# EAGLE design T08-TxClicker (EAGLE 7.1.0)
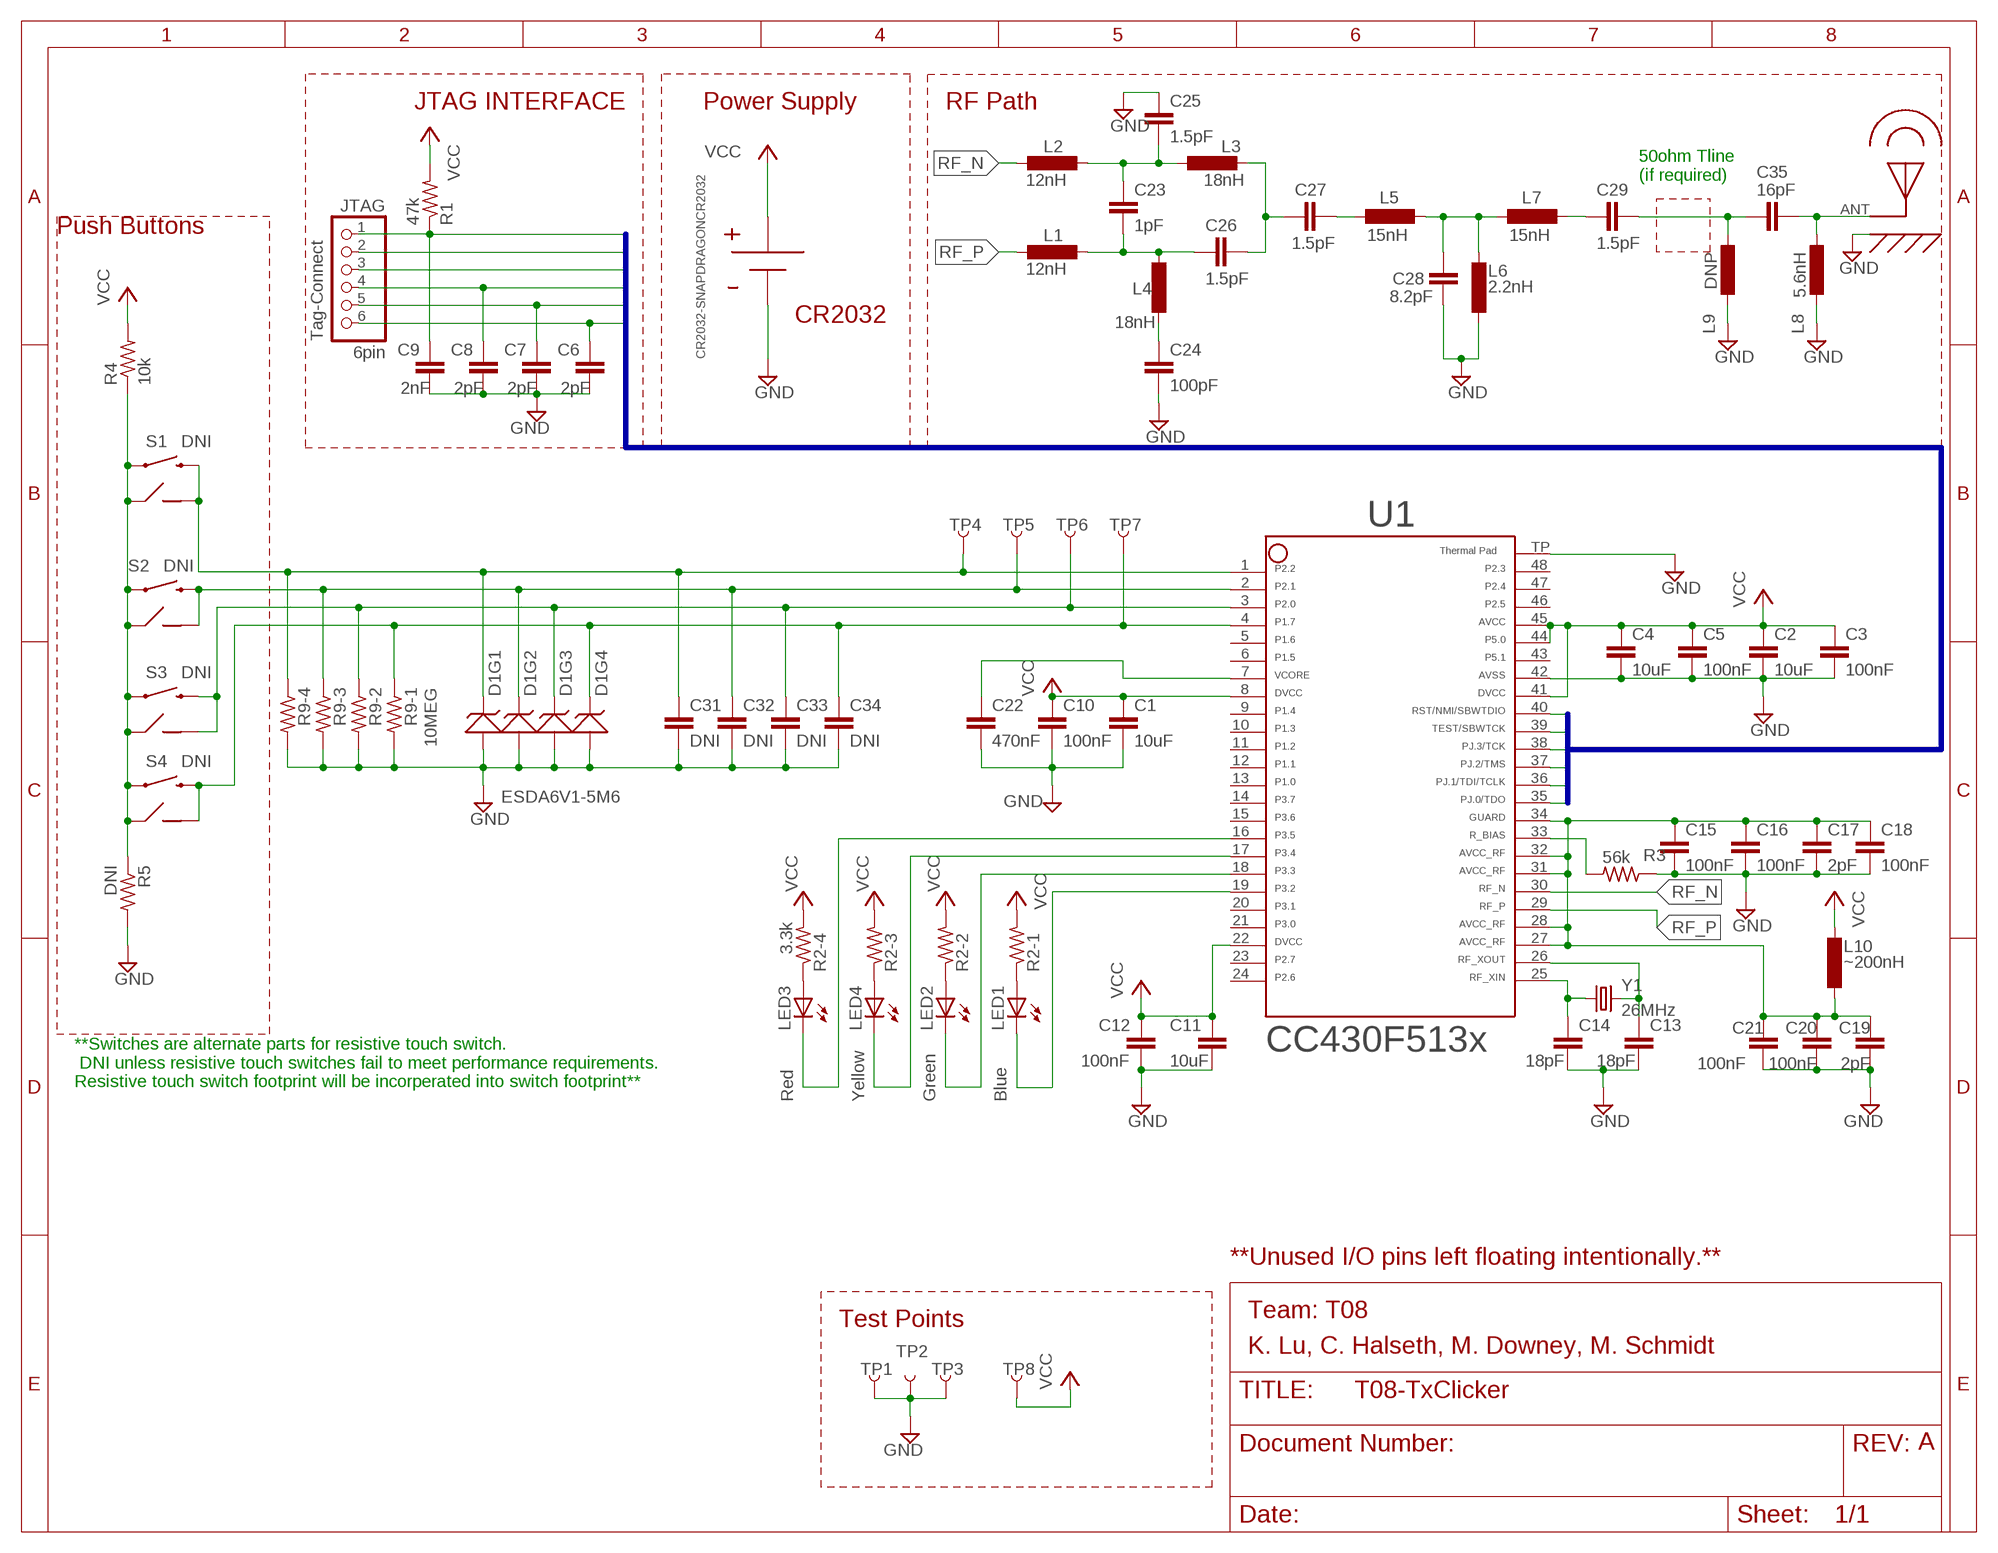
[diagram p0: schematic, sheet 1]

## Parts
C1  10uF  C-EUC0805  [C0805]
C2  10uF  C-EUC0805  [C0805]
C3  100nF  C-EUC0603  [C0603]
C4  10uF  C-EUC0805  [C0805]
C5  100nF  C-EUC0603  [C0603]
C6  2pF  C0603  [C0603]
C7  2pF  C0603  [C0603]
C8  2pF  C0603  [C0603]
C9  2nF  C0603  [C0603]
C10  100nF  C-EUC0603  [C0603]
C11  10uF  C-EUC0805  [C0805]
C12  100nF  C-EUC0603  [C0603]
C13  18pF  C-EUC0402  [C0402]
C14  18pF  C-EUC0402  [C0402]
C15  100nF  C-EUC0603  [C0603]
C16  100nF  C-EUC0603  [C0603]
C17  2pF  C-EUC0603  [C0603]
C18  100nF  C-EUC0603  [C0603]
C19  2pF  C-EUC0603  [C0603]
C20  100nF  C-EUC0603  [C0603]
C21  100nF  C-EUC0603  [C0603]
C22  470nF  C-EUC0603  [C0603]
C23  1pF  C-EUC0402  [C0402]
C24  100pF  C-EUC0402  [C0402]
C25  1.5pF  C-EUC0402  [C0402]
C26  1.5pF  C-EUC0402  [C0402]
C27  1.5pF  C-EUC0402  [C0402]
C28  8.2pF  C-EUC0402  [C0402]
C29  1.5pF  C-EUC0402  [C0402]
C31  DNI  C-EUC0603  [C0603]
C32  DNI  C-EUC0603  [C0603]
C33  DNI  C-EUC0603  [C0603]
C34  DNI  C-EUC0603  [C0603]
C35  16pF  C-EUC0402  [C0402]
D1  ESDA6V1-5M6  [5X-TVS]
JTAG  6pin  PINHD-1X6  [1X06]
L1  12nH  LL0603  [L0603]
L2  12nH  LL0603  [L0603]
L3  18nH  LL0603  [L0603]
L4  18nH  LL0603  [L0603]
L5  15nH  LL0603  [L0603]
L6  2.2nH  LL0603  [L0603]
L7  15nH  LL0603  [L0603]
L8  5.6nH  LL0603  [L0603]
L9  DNP  LL0603  [L0603]
L10  ~200nH  LL0402  [L0402]
LED1  Blue  LEDCHIP-LED0603  [CHIP-LED0603]
LED2  Green  LEDCHIP-LED0603  [CHIP-LED0603]
LED3  Red  LEDCHIP-LED0603  [CHIP-LED0603]
LED4  Yellow  LEDCHIP-LED0603  [CHIP-LED0603]
R1  47k  R-US_R0603  [R0603]
R2  3.3k  R603X42012  [2012(4_RES)]
R3  56k  R-US_R0603  [R0603]
R4  10k  R-US_R0603  [R0603]
R5  DNI  R-US_R0603  [R0603]
R9  10MEG  R603X42012  [2012(4_RES)]
S1  SWITCH-MOMENTARY-212MM  [TACTILE-PTH-12MM]
S2  SWITCH-MOMENTARY-212MM  [TACTILE-PTH-12MM]
S3  SWITCH-MOMENTARY-212MM  [TACTILE-PTH-12MM]
S4  SWITCH-MOMENTARY-212MM  [TACTILE-PTH-12MM]
TP1  TEST-POINT3  [PAD.03X.03]
TP2  TEST-POINT3  [PAD.03X.03]
TP3  TEST-POINT3  [PAD.03X.03]
TP4  TEST-POINT3  [PAD.03X.03]
TP5  TEST-POINT3  [PAD.03X.03]
TP6  TEST-POINT3  [PAD.03X.03]
TP7  TEST-POINT3  [PAD.03X.03]
TP8  TEST-POINT3  [PAD.03X.03]
U1  CC430F513X---RGZ48  [RGZ48]
U$1  TOUCH-PAD  [TOUCH-PAD]
U$2  CR2032-SNAPDRAGONCR2032  [CR2032-SNAPDRAGON]
U$3  TOUCH-PAD  [TOUCH-PAD]
U$4  TOUCH-PAD  [TOUCH-PAD]
U$5  TOUCH-PAD  [TOUCH-PAD]
U$7  PCB_ANTENNA_915MHZOSHP  [PCB_ANTENNA_915MHZ]
Y1  26MHz  CRYSTALTXC-7A  [CRYSTAL-TXC-7A]

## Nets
GND: C1.2 C2.2 C3.2 C4.2 C5.2 C6.2 C7.2 C8.2 C9.2 C10.2 C11.2 C12.2 C13.2 C14.2 C15.2 C16.2 C17.2 C18.2 C19.2 C20.2 C21.2 C22.2 C24.2 C25.1 C28.1 C31.2 C32.2 C33.2 C34.2 D1.2 L6.2 L8.1 L9.1 R3.1 R5.2 R9.2 R9.4 R9.6 R9.8 TP1.P$1 TP2.P$1 TP3.P$1 U1.42 U1.TP U$2.V- U$7.GPLANE
N$1: C23.2 C26.2 L1.1 L4.1
N$2: C23.1 C25.2 L2.1 L3.2
N$3: C26.1 C27.1 L3.1
N$4: C24.1 L4.2
N$5: C27.2 L5.1
N$6: C28.2 L5.2 L6.1 L7.1
N$7: C29.1 C35.2 L9.2
N$8: C29.2 L7.2
N$9: C15.1 C16.1 C17.1 C18.1 C19.1 C20.1 C21.1 L10.P$2 U1.27 U1.28 U1.31 U1.32 U1.34
N$10: C35.1 L8.2 U$7.ANT
N$18: LED1.A R2.1
N$20: R4.1 R5.1 S1.1 S2.1 S3.1 S4.1 U$1.P$1 U$1.P$2 U$1.P$3 U$1.P$4 U$3.P$1 U$3.P$2 U$3.P$3 U$3.P$4 U$4.P$1 U$4.P$2 U$4.P$3 U$4.P$4 U$5.P$1 U$5.P$2 U$5.P$3 U$5.P$4
N$21: LED3.A R2.7
N$23: LED4.A R2.5
N$24: LED2.A R2.3
P1.7: C34.1 D1.5 R9.1 S4.3 TP7.P$1 U1.4 U$1.VCC
P2.0: C33.1 D1.4 R9.3 S3.3 TP6.P$1 U1.3 U$3.VCC
P2.1: C32.1 D1.3 R9.5 S2.3 TP5.P$1 U1.2 U$4.VCC
P2.2: C31.1 D1.1 R9.7 S1.3 TP4.P$1 U1.1 U$5.VCC
P3.2: LED1.C U1.19
P3.3: LED2.C U1.18
P3.4: LED4.C U1.17
P3.5: LED3.C U1.16
PJ.0/TDO: C6.1 JTAG.6 U1.35
PJ.1/TDI/TCLK: C7.1 JTAG.5 U1.36
PJ.2/TMS: C8.1 JTAG.4 U1.37
PJ.3/TCK: JTAG.3 U1.38
R_BIAS: R3.2 U1.33
RF_N: L2.2 U1.30
RF_P: L1.2 U1.29
RF_XIN: C14.1 U1.25 Y1.P$1
RF_XOUT: C13.1 U1.26 Y1.P$2
RST/NMI/SBWTDIO: C9.1 JTAG.1 R1.1 U1.40
TEST/SBWTCK: JTAG.2 U1.39
VCC: C1.1 C2.1 C3.1 C4.1 C5.1 C10.1 C11.1 C12.1 L10.P$1 R1.2 R2.2 R2.4 R2.6 R2.8 R4.2 TP8.P$1 U1.8 U1.22 U1.41 U1.44 U1.45 U$2.V+
VCORE: C22.1 U1.7
Unconnected: D1.6 U1.5 U1.6 U1.9 U1.10 U1.11 U1.12 U1.13 U1.14 U1.15 U1.20 U1.21 U1.23 U1.24 U1.43 U1.46 U1.47 U1.48

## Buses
PJ.0/TDO,PJ.1/TDI/TCLK,PJ.2/TMS,PJ.3/TCK,TEST/SBWTCK,RST/NMI/SBWTDIO

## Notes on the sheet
- JTAG INTERFACE | Power Supply | RF Path
- 50ohm Tline
  (if required)
- Push Buttons
- CR2032
- Tag-Connect
- DNI
- DNI
- DNI
- DNI
- **Switches are alternate parts for resistive touch switch.
   DNI unless resistive touch switches fail to meet performance requirements.
  Resistive touch switch footprint will be incorperated into switch footprint**
- **Unused I/O pins left floating intentionally.**
- Team: T08
- Team: T08 | Team: T08 | Team: T08 | Team: T08
- Test Points
- K. Lu, C. Halseth, M. Downey, M. Schmidt
- A

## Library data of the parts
C1-C5 C10-C29 C31-C35 = rcl:C-EU: CAPACITOR, European symbol
C6-C9 = rcl-amber:C
D1 = TVS:ESDA6V1-5M6
JTAG = adafruit:PINHD-1X6: PIN HEADER
L1-L10 = rcl-amber:L
LED1-LED4 = adafruit:LED: LED
R1 R3-R5 = rcl:R-US_: RESISTOR, American symbol
R2 R9 = QuadResistor:R603X4: Quad resistor package 0603
S1-S4 = SparkFun-Electromechanical:SWITCH-MOMENTARY-2: Various NO switches- pushbuttons, reed, etc; PROD_ID: SWCH-09185
TP1-TP8 = SparkFun-Passives:TEST-POINT: Bare copper test points for troubleshooting or ICT
U1 = TI_MSP430_v16_truncated:CC430F513X---RGZ48: ***CC430F513X***RGZ48 ** ** Rev 1.0 ** 06/2010 * http://focus.ti.com/docs/prod/folders/print/cc430f5137.html
U$1 U$3-U$5 = TouchPad:TOUCH-PAD
U$2 = CR2032-SnapDragon:CR2032-SNAPDRAGON: HOLDER SNAP DRAGON CR2032 SMD
U$7 = PCB_Antenna_915MHz-halseth:PCB_ANTENNA_915MHZ
Y1 = SparkFun-FreqCtrl:CRYSTAL: Various standard crystals. Proven footprints. Spark Fun Electronics SKU : COM-00534

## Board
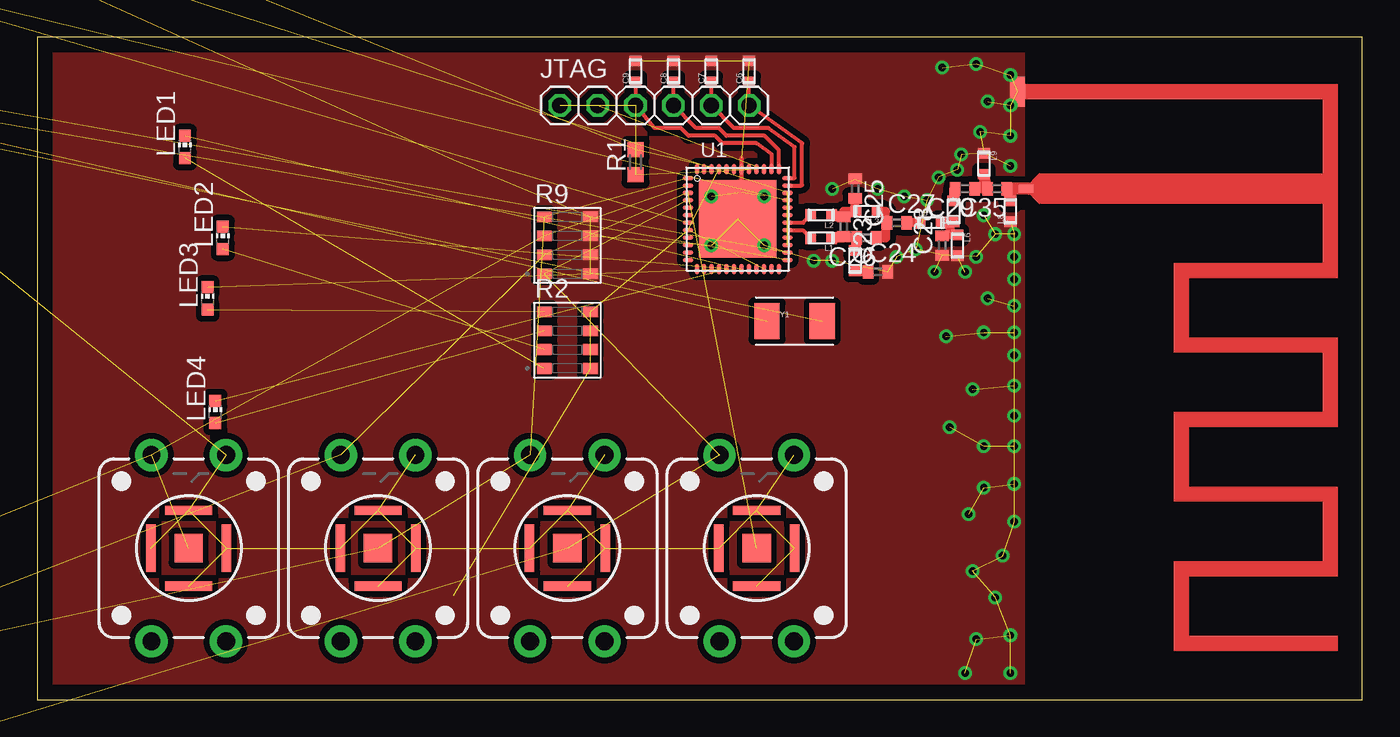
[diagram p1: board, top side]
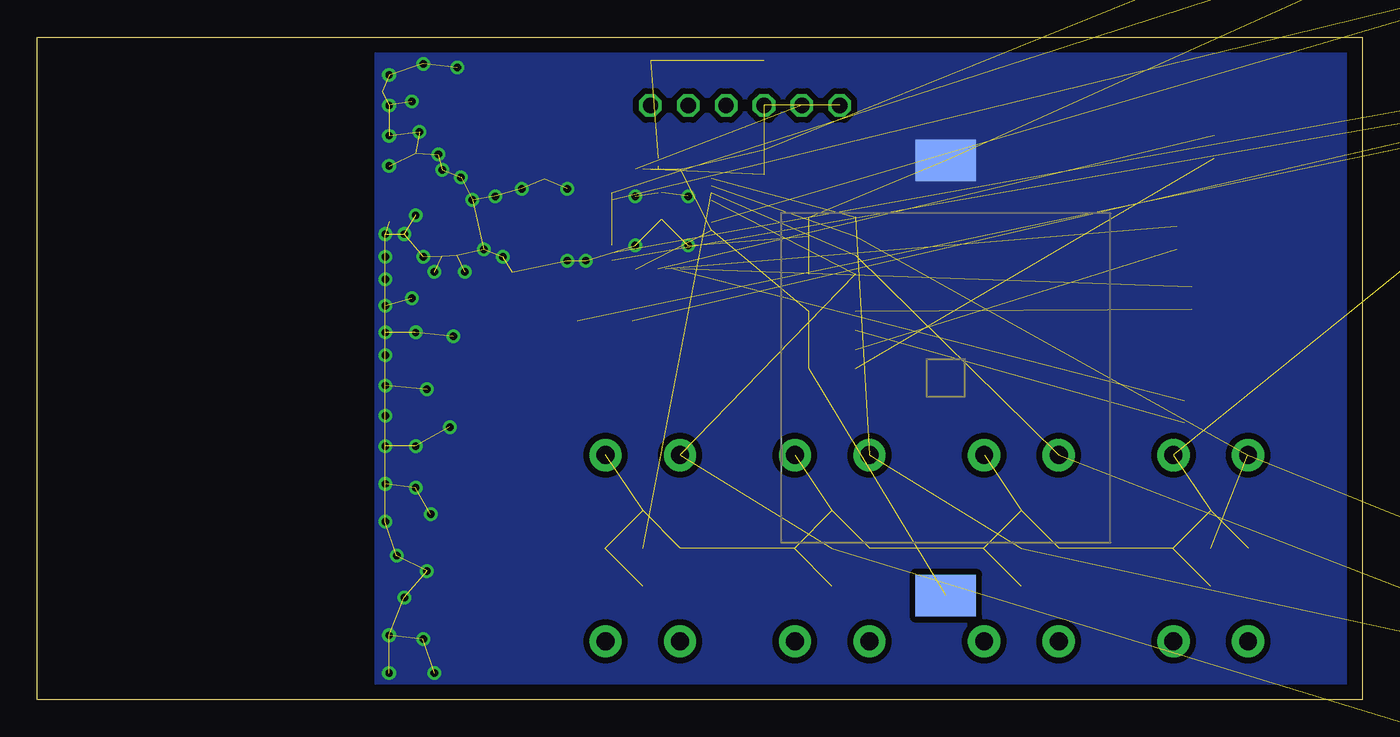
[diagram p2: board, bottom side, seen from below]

Size 88.88 x 44.45 mm. Coordinates in mm from the lower left corner, seen from the top.
Outline: 0,0 88.88,0 88.88,44.45 0,44.45 0,0
Copper layers (1*16): Top 0.035mm / dielectric 1.5mm / Bottom 0.035mm
Design rules "default": minimum track width 10mil, minimum drill 24mil, track to track 8mil, track to pad 8mil, pad to pad 8mil, via to via 8mil, smd to smd 8mil, copper to edge 40mil, drill to drill 8mil, minimum pad ring 10mil, minimum via ring 8mil, stop-mask expansion 4mil, vias tented up to drill 0mil, thermal gap 10mil

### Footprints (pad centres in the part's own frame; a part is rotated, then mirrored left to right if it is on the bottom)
C0805 = smd 1.3 x 1.5: 1 -0.95,0; 2 0.95,0
C0603 = smd 1.1 x 1: 1 -0.85,0; 2 0.85,0
C0603' = smd 0.7 x 0.8: 1 -0.7,0; 2 0.7,0
C0402 = smd 0.7 x 0.9: 1 -0.65,0; 2 0.65,0
5X-TVS = smd 0.254 x 0.66: 1 -0.508,-0.483; 2 0,-0.483; 3 0.508,-0.483; 4 0.508,0.483; 5 0,0.483; 6 -0.508,0.483
1X06 = drill 1.016 octagon: 1 -6.35,0; 2 -3.81,0; 3 -1.27,0; 4 1.27,0; 5 3.81,0; 6 6.35,0
L0603 = smd 0.7 x 0.8: 1 -0.7,0; 2 0.7,0
L0402 = smd 0.5 x 0.5: P$1 -0.5,0; P$2 0.5,0
CHIP-LED0603 = smd 0.8 x 0.8: A 0,-0.75; C 0,0.75
R0603 = smd 1 x 1.1: 1 -0.85,0; 2 0.85,0
2012(4_RES) = smd 1 x 0.71: 1 -1.55,-1.905; 2 1.55,-1.905; 3 -1.55,-0.635; 4 1.55,-0.635; 5 -1.55,0.635; 6 1.55,0.635; 7 -1.55,1.905; 8 1.55,1.905
TACTILE-PTH-12MM = drill 1.2 pad 2.159: 1 6.25,-2.5; 2 -6.25,-2.5; 3 6.25,2.5; 4 -6.25,2.5
PAD.03X.03 = smd 0.762 x 0.762: P$1 0,0
RGZ48 = smd 0.7 x 0.3: 1 -3.35,2.75; 2 -3.35,2.25; 3 -3.35,1.75; 4 -3.35,1.25; 5 -3.35,0.75; 6 -3.35,0.25; 7 -3.35,-0.25; 8 -3.35,-0.75; 9 -3.35,-1.25; 10 -3.35,-1.75; 11 -3.35,-2.25; 12 -3.35,-2.75; 25 3.35,-2.75; 26 3.35,-2.25; 27 3.35,-1.75; 28 3.35,-1.25; 29 3.35,-0.75; 30 3.35,-0.25; 31 3.35,0.25; 32 3.35,0.75; 33 3.35,1.25; 34 3.35,1.75; 35 3.35,2.25; 36 3.35,2.75 | smd 0.3 x 0.7: 13 -2.75,-3.35; 14 -2.25,-3.35; 15 -1.75,-3.35; 16 -1.25,-3.35; 17 -0.75,-3.35; 18 -0.25,-3.35; 19 0.25,-3.35; 20 0.75,-3.35; 21 1.25,-3.35; 22 1.75,-3.35; 23 2.25,-3.35; 24 2.75,-3.35; 37 2.75,3.35; 38 2.25,3.35; 39 1.75,3.35; 40 1.25,3.35; 41 0.75,3.35; 42 0.25,3.35; 43 -0.25,3.35; 44 -0.75,3.35; 45 -1.25,3.35; 46 -1.75,3.35; 47 -2.25,3.35; 48 -2.75,3.35 | smd 5.2 x 5.2: TP 0,0
TOUCH-PAD = smd 3.175 x 0.635: P$1 0,2.54; P$3 0,-2.54 | smd 0.635 x 3.175: P$2 2.54,0; P$4 -2.54,0 | smd 1.905 x 1.905: VCC 0,0
CR2032-SNAPDRAGON = smd 2.794 x 4.064: V+ 14.605,0; V- -14.605,0
PCB_ANTENNA_915MHZ = smd 0.5 x 1: ANT 0,-0.9 | smd 2 x 1: GPLANE -6.51,-1.5
CRYSTAL-TXC-7A = smd 1.7 x 2.4: P$1 1.85,0; P$2 -1.85,0

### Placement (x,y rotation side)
C1  not placed on the board
C2  not placed on the board
C3  not placed on the board
C4  not placed on the board
C5  not placed on the board
C6  2pF  [C0603']  47.75,42.16 90 top
C7  2pF  [C0603']  45.21,42.16 90 top
C8  2pF  [C0603']  42.67,42.16 90 top
C9  2nF  [C0603']  40.13,42.16 90 top
C10  not placed on the board
C11  not placed on the board
C12  not placed on the board
C13  not placed on the board
C14  not placed on the board
C15  not placed on the board
C16  not placed on the board
C17  not placed on the board
C18  not placed on the board
C19  not placed on the board
C20  not placed on the board
C21  not placed on the board
C22  not placed on the board
C23  54.1,31.75 270 top
C24  56.39,28.7 0 top
C25  54.86,34.29 270 top
C26  55.63,30.99 180 top
C27  57.66,32 0 top
C28  60.71,30.48 90 top
C29  62.23,34.29 180 top
C31  not placed on the board
C32  not placed on the board
C33  not placed on the board
C34  not placed on the board
C35  64.39,34.29 180 top
D1  not placed on the board
JTAG  41.4,39.88 0 top
L1  52.58,30.99 180 top
L2  52.58,32.51 180 top
L3  55.63,32.77 180 top
L4  54.86,29.46 270 top
L5  59.94,32 0 top
L6  61.72,30.48 270 top
L7  61.47,32.77 90 top
L8  65.28,32.77 90 top
L9  63.5,35.97 270 top
L10  not placed on the board
LED1  9.91,37.08 0 top
LED2  12.45,30.99 0 top
LED3  11.43,26.92 0 top
LED4  11.94,19.3 0 top
R1  40.13,36.07 90 top
R2  35.56,24.13 0 top
R3  not placed on the board
R4  not placed on the board
R5  not placed on the board
R9  35.56,30.48 0 top
S1  35.56,10.16 90 top
S2  10.16,10.16 90 top
S3  22.86,10.16 90 top
S4  48.26,10.16 90 top
TP1  not placed on the board
TP2  not placed on the board
TP3  not placed on the board
TP4  not placed on the board
TP5  not placed on the board
TP6  not placed on the board
TP7  not placed on the board
TP8  not placed on the board
U1  46.99,32.26 0 top
U$1  35.56,10.16 0 top
U$2  27.94,21.59 270 bottom
U$3  48.26,10.16 0 top
U$4  10.16,10.16 0 top
U$5  22.86,10.16 0 top
U$7  67.23,34.29 270 top
Y1  50.8,25.4 0 top

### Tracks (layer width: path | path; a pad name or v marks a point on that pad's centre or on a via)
GND  (via drill 0.5)  (99 unrouted)
  Top 0.305: U1.42 47.24,34.04 46.99,34.04 U1.TP | 47.24,36.32 47.24,35.81
  other vias: 48.77,33.78 45.21,33.78 45.21,30.48 48.77,30.48 64.26,6.86 60.71,42.42 62.99,42.67 65.28,41.91 63.75,40.13 65.28,39.88 65.28,37.85 63.25,38.1 61.98,36.58 61.72,35.56 60.45,35.05 59.69,33.53 58.17,33.78 56.39,34.29 53.34,34.29 53.34,29.46 52.07,29.46 57.66,29.72 58.93,30.23 60.2,28.7 62.23,28.7 62.99,29.72 63.5,32.51 64.26,31.24 65.53,31.24 65.53,29.72 65.53,28.19 63.75,26.92 65.53,26.42 65.28,35.81 63.5,24.64 60.96,24.38 65.53,24.64 65.53,23.11 65.53,21.08 62.74,20.83 61.21,18.29 63.5,17.02 65.53,17.02 65.53,19.05 65.53,14.48 63.5,14.22 62.48,12.45 65.53,11.94 64.77,9.65 62.74,8.64 62.99,4.06 65.28,4.32 65.28,1.78 62.23,1.78
  pour Bottom (isolate 0.406, no thermals): 0,44.45 0,0 66.04,0 66.04,44.45
  pour Top (isolate 0.406, no thermals): 0,44.45 66.04,44.45 66.04,0 0,0
N$1
  Top 0.61: 54.1,30.99 C26.2 54.93,30.16 L4.1 | L1.1 54.1,30.99 | 54.1,30.99 C23.2
N$2
  Top 0.61: C25.2 54.86,32.77 L3.2 54.1,32.77 C23.1 54.1,32.51 L2.1
N$3
  Top 0.61: C27.1 56.9,32 | 56.9,32 56.9,32.77 L3.1 | 56.9,32 56.9,30.99 C26.1
N$4
  Top 0.61: C24.1 54.86,28.7 L4.2
N$5
  Top 0.61: L5.1 C27.2
N$6
  Top 0.61: L6.1 61.21,31.18 | 61.21,31.18 C28.2 | 61.21,31.18 61.21,32.07 L7.1 61.47,32 L5.2
N$7
  Top 0.61: L9.2 63.54,35.27 C35.2 C29.1
N$8
  Top 0.61: C29.2 61.47,34.29 L7.2
N$9  (12 unrouted)
N$10
  Top 0.61: U$7.ANT 65.53,34.29 | 65.28,34.29 C35.1 65.24,33.47 L8.2
  Top 0.813: 66.55,34.29 65.53,34.29 65.28,34.29 65.28,33.53
N$11
  Top 0.61: 63.5,34.29 63.5,35.05
N$18  (1 unrouted)
N$20  (21 unrouted)
N$21  (1 unrouted)
N$23  (1 unrouted)
N$24  (1 unrouted)
P1.7  (6 unrouted)
P2.0  (6 unrouted)
P2.1  (6 unrouted)
P2.2  (6 unrouted)
P3.2  (1 unrouted)
P3.3  (1 unrouted)
P3.4  (1 unrouted)
P3.5  (1 unrouted)
PJ.0/TDO
  Top 0.254: U1.35 51.27,34.51 51.31,34.54 51.31,37.34 JTAG.6 C6.1
PJ.1/TDI/TCLK
  Top 0.254: U1.36 50.8,35.01 50.8,37.08 49.02,38.35 46.74,38.35 JTAG.5 C7.1
PJ.2/TMS
  Top 0.254: U1.37 49.74,36.87 48.77,37.85 46.23,37.85 45.72,38.35 44.2,38.35 JTAG.4 C8.1
PJ.3/TCK
  Top 0.254: U1.38 49.28,35.61 49.28,36.58 48.26,37.34 45.97,37.34 45.47,37.85 43.69,37.85 43.18,38.35 41.4,38.35 JTAG.3
R_BIAS  (1 unrouted)
RF_N
  Top 0.254: U1.30 51.37,32.01 L2.2
RF_P
  Top 0.254: U1.29 51.36,31.51 L1.2
RF_XIN  (2 unrouted)
RF_XOUT  (2 unrouted)
RST/NMI/SBWTDIO  (3 unrouted)
  Top 0.254: C9.1 40.13,39.88
TEST/SBWTCK  (1 unrouted)
VCC  (21 unrouted)
VCORE  (1 unrouted)

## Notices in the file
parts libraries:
SparkFun-Electromechanical: Licensing: CC v3.0 Share-Alike You are welcome to use this library for commercial purposes.
